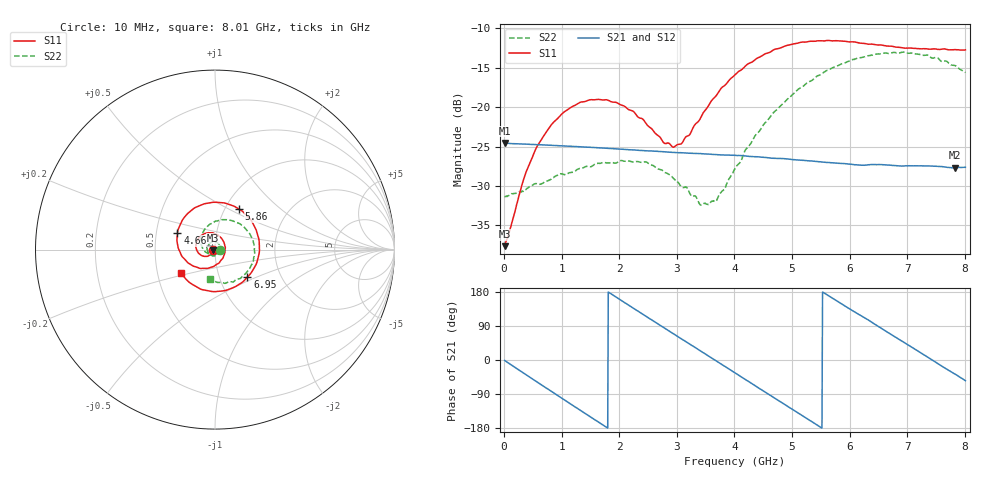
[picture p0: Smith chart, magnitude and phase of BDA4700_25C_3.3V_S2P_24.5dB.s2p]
!Agilent Technologies,E5071B,MY42404982,A.09.10
!Date: Mon Oct 20 18:13:22 2025
!Data & Calibration Information:
!Freq	S11:SOLT2(ON)	S21:SOLT2(ON)	S12:SOLT2(ON)	S22:SOLT2(ON)
# Hz S RI R 50
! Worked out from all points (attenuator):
!   801 points, 10 MHz to 8.01 GHz, reference 50 ohm
!   highest |S21| = -24.56 dB at 10 MHz (marker M1); lowest = -27.7 dB at 7.83 GHz (marker M2)
!   lowest |S11| = -37.7 dB at 10 MHz (marker M3), VSWR 1.03, Z = 48.7 - j0.141 ohm
!   |S11| at or under -10 dB: start of sweep to end of sweep
!   |S22| runs from -32.4 to -13.0 dB; largest |S21 - S12| = 0.00066
!   S11 on the Smith chart (normalised r, x): 10 MHz: 0.97, -0.00; 4.66 GHz: 0.64, +0.13; 5.86 GHz: 1.17, +0.56; 6.95 GHz: 1.36, -0.44; 8.01 GHz: 0.66, -0.18
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1e7  -0.013 -0.00144  0.0591 -0.00124  0.0591 -0.00131  0.0271 -0.000808
3.5e8  -0.0239 -0.0264  0.0473 -0.0339  0.0473 -0.0339  0.0229 -0.0184
5.8e8  -0.0429 -0.0374  0.0301 -0.0493  0.03 -0.0494  0.0145 -0.0292
1e9  -0.0868 -0.0243  -0.0104 -0.0559  -0.0104 -0.0559  -0.0146 -0.0348
1.35e9  -0.1068 0.0158  -0.0398 -0.0394  -0.0398 -0.0394  -0.0366 -0.0183
1.97e9  -0.0568 0.0898  -0.0521 0.0154  -0.0521 0.0153  -0.0348 0.028
2.45e9  0.0204 0.0776  -0.0238 0.0472  -0.0238 0.0472  -0.00322 0.0449
2.68e9  0.0479 0.045  -0.00408 0.0522  -0.00413 0.0522  0.0131 0.0382
2.93e9  0.0557 -0.00134  0.0174 0.0486  0.0173 0.0485  0.0252 0.0252
3.06e9  0.0516 -0.027  0.0275 0.0434  0.0271 0.0436  0.028 0.0154
3.43e9  0.000758 -0.0882  0.0469 0.019  0.0469 0.0191  0.0201 -0.013
3.69e9  -0.0579 -0.1041  0.0499 -0.00255  0.0499 -0.00267  0.00144 -0.0255
4.01e9  -0.1379 -0.0817  0.041 -0.0277  0.0411 -0.0275  -0.0313 -0.026
4.66e9  -0.209 0.0927  -0.00583 -0.047  -0.00565 -0.0471  -0.0792 0.0438
5.35e9  -0.0511 0.2568  -0.0436 -0.013  -0.0435 -0.0132  -0.0158 0.147
5.86e9  0.1349 0.2252  -0.0373 0.0231  -0.0373 0.0231  0.0978 0.1607
6.27e9  0.2318 0.1021  -0.0151 0.0401  -0.0146 0.0402  0.1833 0.1014
6.68e9  0.2365 -0.06  0.0139 0.0405  0.0139 0.0405  0.2191 0.000157
6.95e9  0.1809 -0.1529  0.0293 0.0305  0.0294 0.0304  0.2108 -0.0735
7.42e9  0.0112 -0.2331  0.0423 0.000981  0.0422 0.000933  0.123 -0.1648
7.83e9  -0.1436 -0.1822  0.0328 -0.0249  0.0328 -0.025  0.0133 -0.1831
8.01e9  -0.1917 -0.1288  0.024 -0.0338  0.0241 -0.0337  -0.0305 -0.1629
